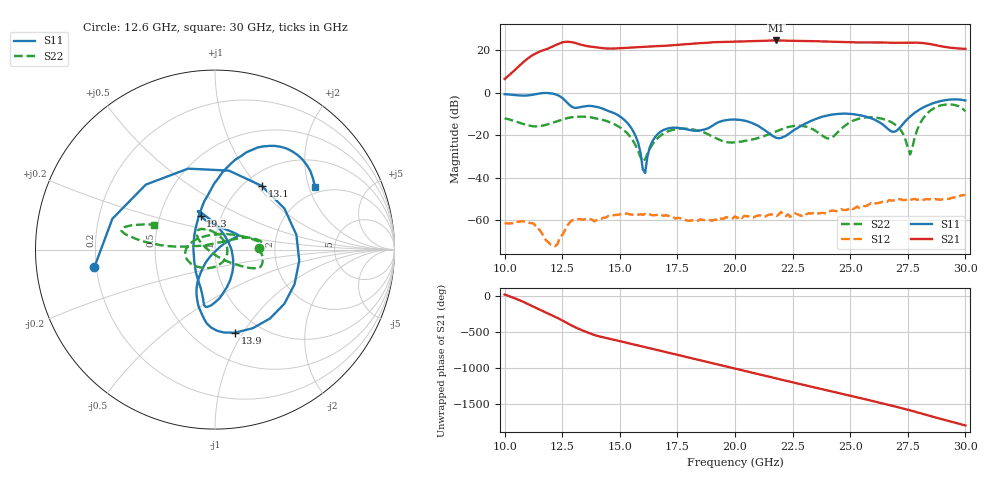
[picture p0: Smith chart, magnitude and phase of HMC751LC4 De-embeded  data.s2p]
! Hittite Microwave Corp
! Chelmsford, MA 01824
! http://www.hittite.com
! Tel: 978-250-3343
! Fax: 978-250-3373
! Device  :  HMC751LC4
! Description:  SMT PHEMT LOW NOISE AMPLIFIER
! Frequency  :  17 GHz - 27 GHz
! Package  : LC4  - 4x4 mm QFN Ceramic High frequency SMT Package: 24 pin
! Ports  :  2 RF, 3 DC
!  Pin  4  = Rfin  = Port 1
!  Pin  15  = Rfout = Port 2
!  pin  22 = VDD1
!  Pin  21  = VDD2
!  PIN  20  = VDD3
! Voltages:  Vdd  =  5.0 Volts
! Currents :  Idd  = 80.0 mA
! Data:  The device was measured on evaluation board 123813-1.
!  Data was collected using a calibrated network analyzer.
!  The evaluation circuit board was modeled and simulated.This was use
!  to removed the evaluation board circuit from the measured data.
!  The reference plane is the center of the package pin.
! Misc:  Lot #
!Date Measured:  08 - 12 -2009
! Date:  08 - 13 -2009
! Note:
!  Hittite Microwave supplies this data as a sample of measured data at the
!  package pin for this package product.  Your particular data for this product
!  may vary.
!  Data was taken at 25 degrees C.
!  Hittite Microwave reserves the right to change this data at anytime.
# MHz S MA R 50
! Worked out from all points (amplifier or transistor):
!   201 points, 10 GHz to 30 GHz, reference 50 ohm
!   highest |S21| = 24.6 dB at 21.8 GHz (marker M1)
!   |S21| within 3 dB of that: 16.06 GHz to 29.09 GHz (13.04 GHz wide, 57.8 % of centre)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
!   unconditionally stable (mu >= 1): start of sweep to end of sweep
!   at 13.3 GHz: K = 25.29, MAG = 24.1 dB, |S12| = -59.5 dB
!   at 20 GHz: K = 23.88, MAG = 24.3 dB, |S12| = -58.2 dB
!   at 30 GHz: K = 5.91, MAG = 23.7 dB, |S12| = -48.1 dB
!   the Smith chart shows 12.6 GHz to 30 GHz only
!   S11 on the Smith chart (normalised r, x): 12.6 GHz: 0.19, -0.07; 13.1 GHz: 1.20, +1.06; 13.9 GHz: 0.77, -0.92; 19.3 GHz: 0.80, +0.31; 30 GHz: 1.78, +2.20
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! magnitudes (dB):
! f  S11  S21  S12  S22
! 10 GHz  -0.6  6.5  -61.5  -12.0
! 11.2 GHz  -0.9  17.6  -61.3  -15.7
! 12.2 GHz  -0.7  22.4  -72.2  -13.7
! 12.6 GHz  -3.4  23.9  -65.1  -12.3
! 13.1 GHz  -7.1  23.4  -59.4  -11.3
! 13.4 GHz  -6.5  22.4  -59.8  -11.2
! 13.9 GHz  -6.4  21.5  -60.5  -11.9
! 15.4 GHz  -15.1  21.2  -57.1  -20.0
! 16.1 GHz  -37.8  21.7  -57.0  -31.3
! 16.3 GHz  -25.7  21.8  -57.3  -26.4
! 16.7 GHz  -18.9  22.0  -57.4  -20.8
! 19.3 GHz  -13.8  23.9  -58.7  -22.0
! 20 GHz  -12.6  24.1  -58.2  -23.3
! 21.8 GHz  -21.2  24.6  -58.0  -18.2
! 23.4 GHz  -12.8  24.3  -56.7  -17.3
! 24.1 GHz  -10.5  24.1  -55.9  -21.5
! 25.2 GHz  -10.2  23.7  -54.4  -12.8
! 26.7 GHz  -17.5  23.6  -50.5  -13.4
! 27.6 GHz  -11.2  23.6  -50.6  -29.1
! 28 GHz  -8.0  23.6  -50.3  -15.1
! 28.5 GHz  -5.3  22.9  -50.1  -8.2
! 30 GHz  -3.6  20.7  -48.1  -8.7
